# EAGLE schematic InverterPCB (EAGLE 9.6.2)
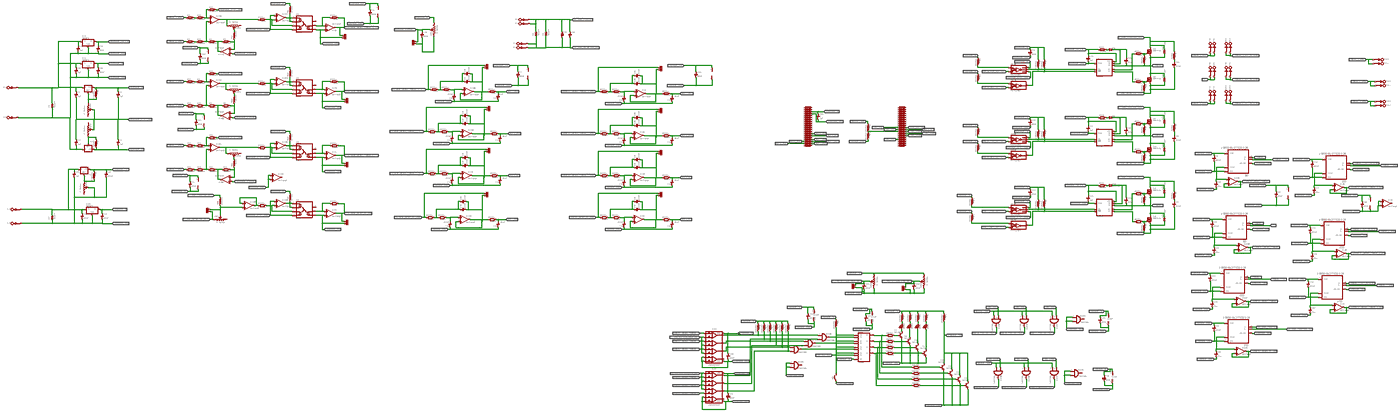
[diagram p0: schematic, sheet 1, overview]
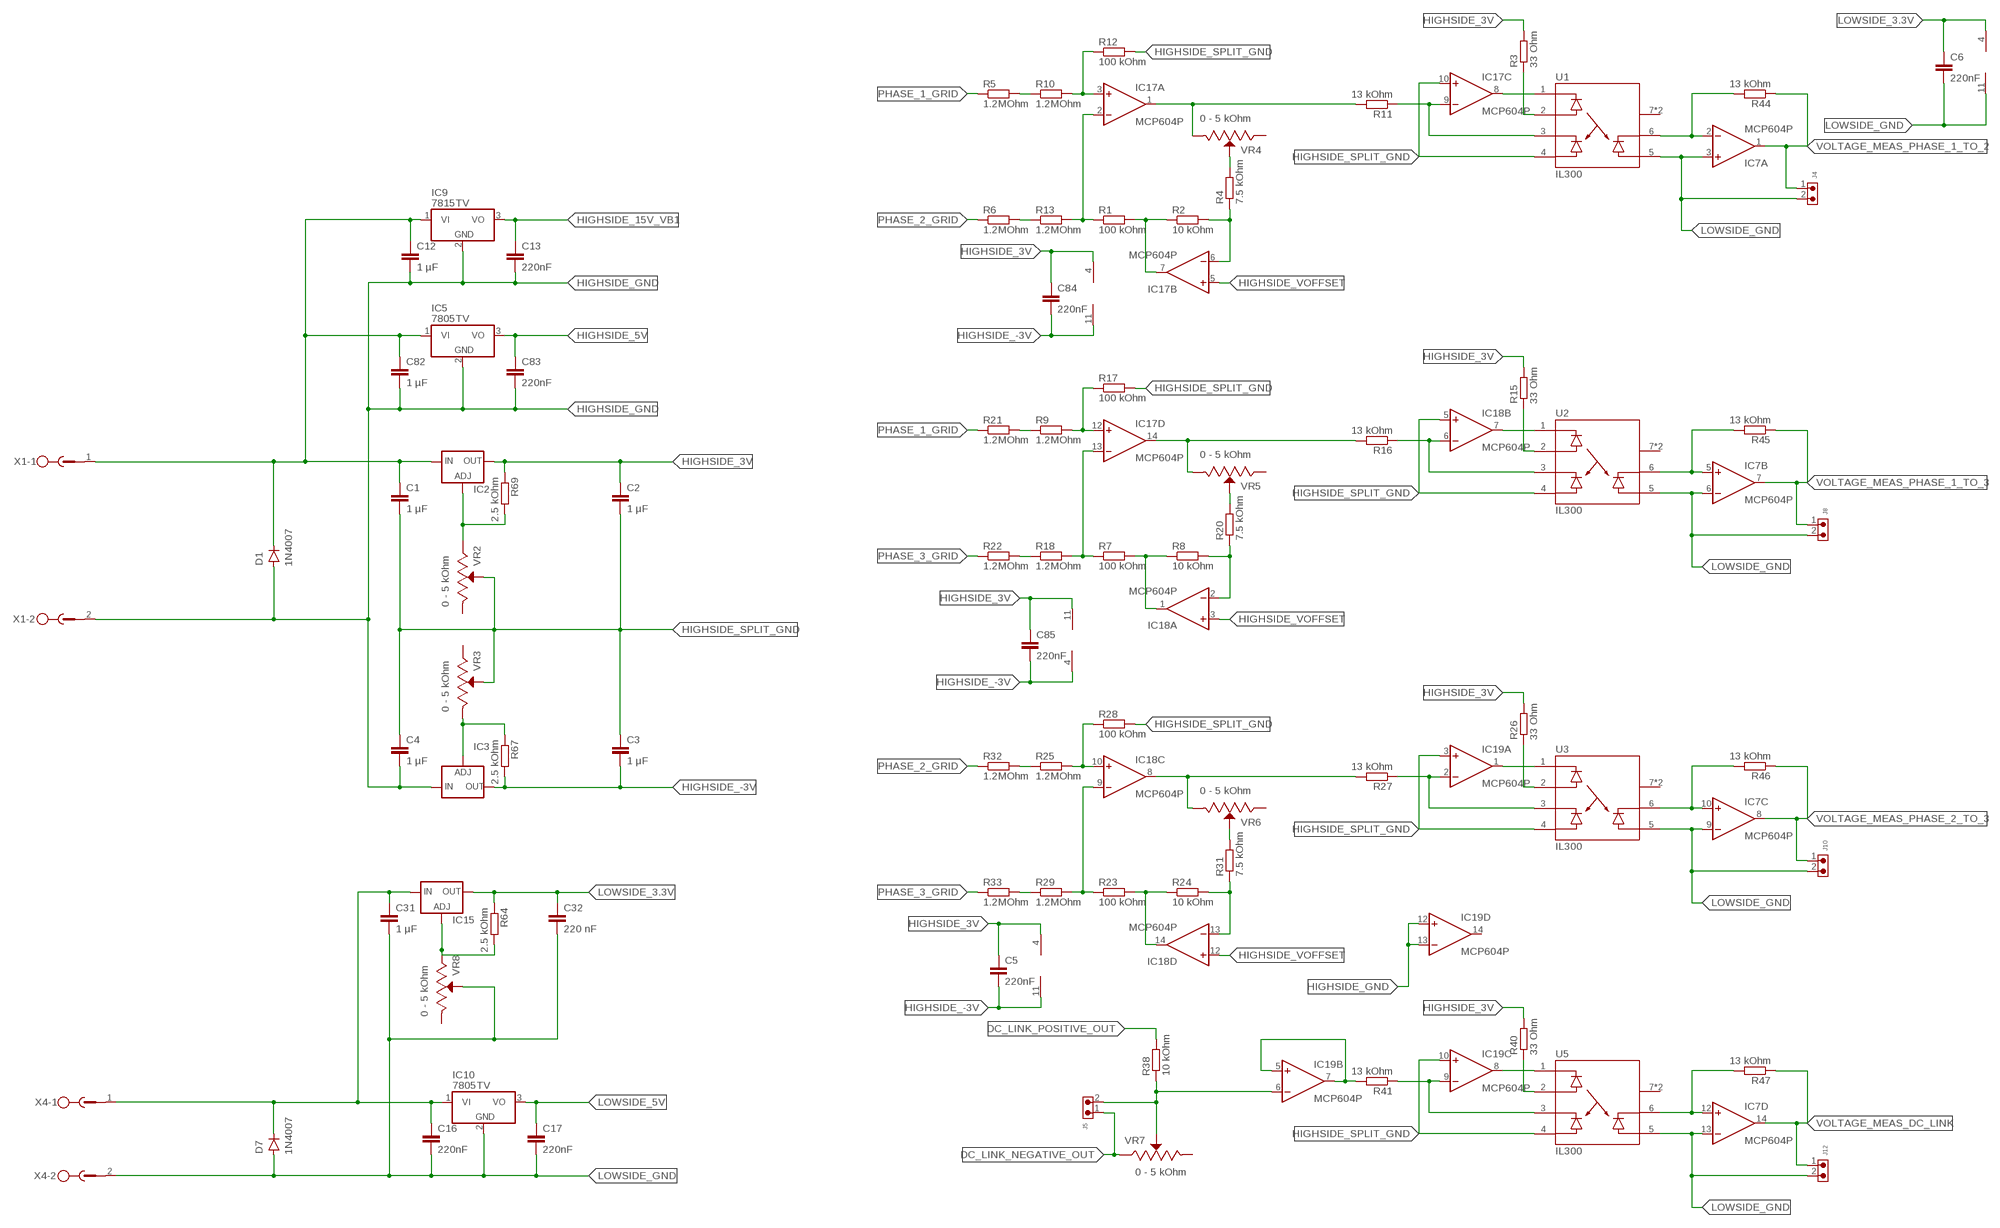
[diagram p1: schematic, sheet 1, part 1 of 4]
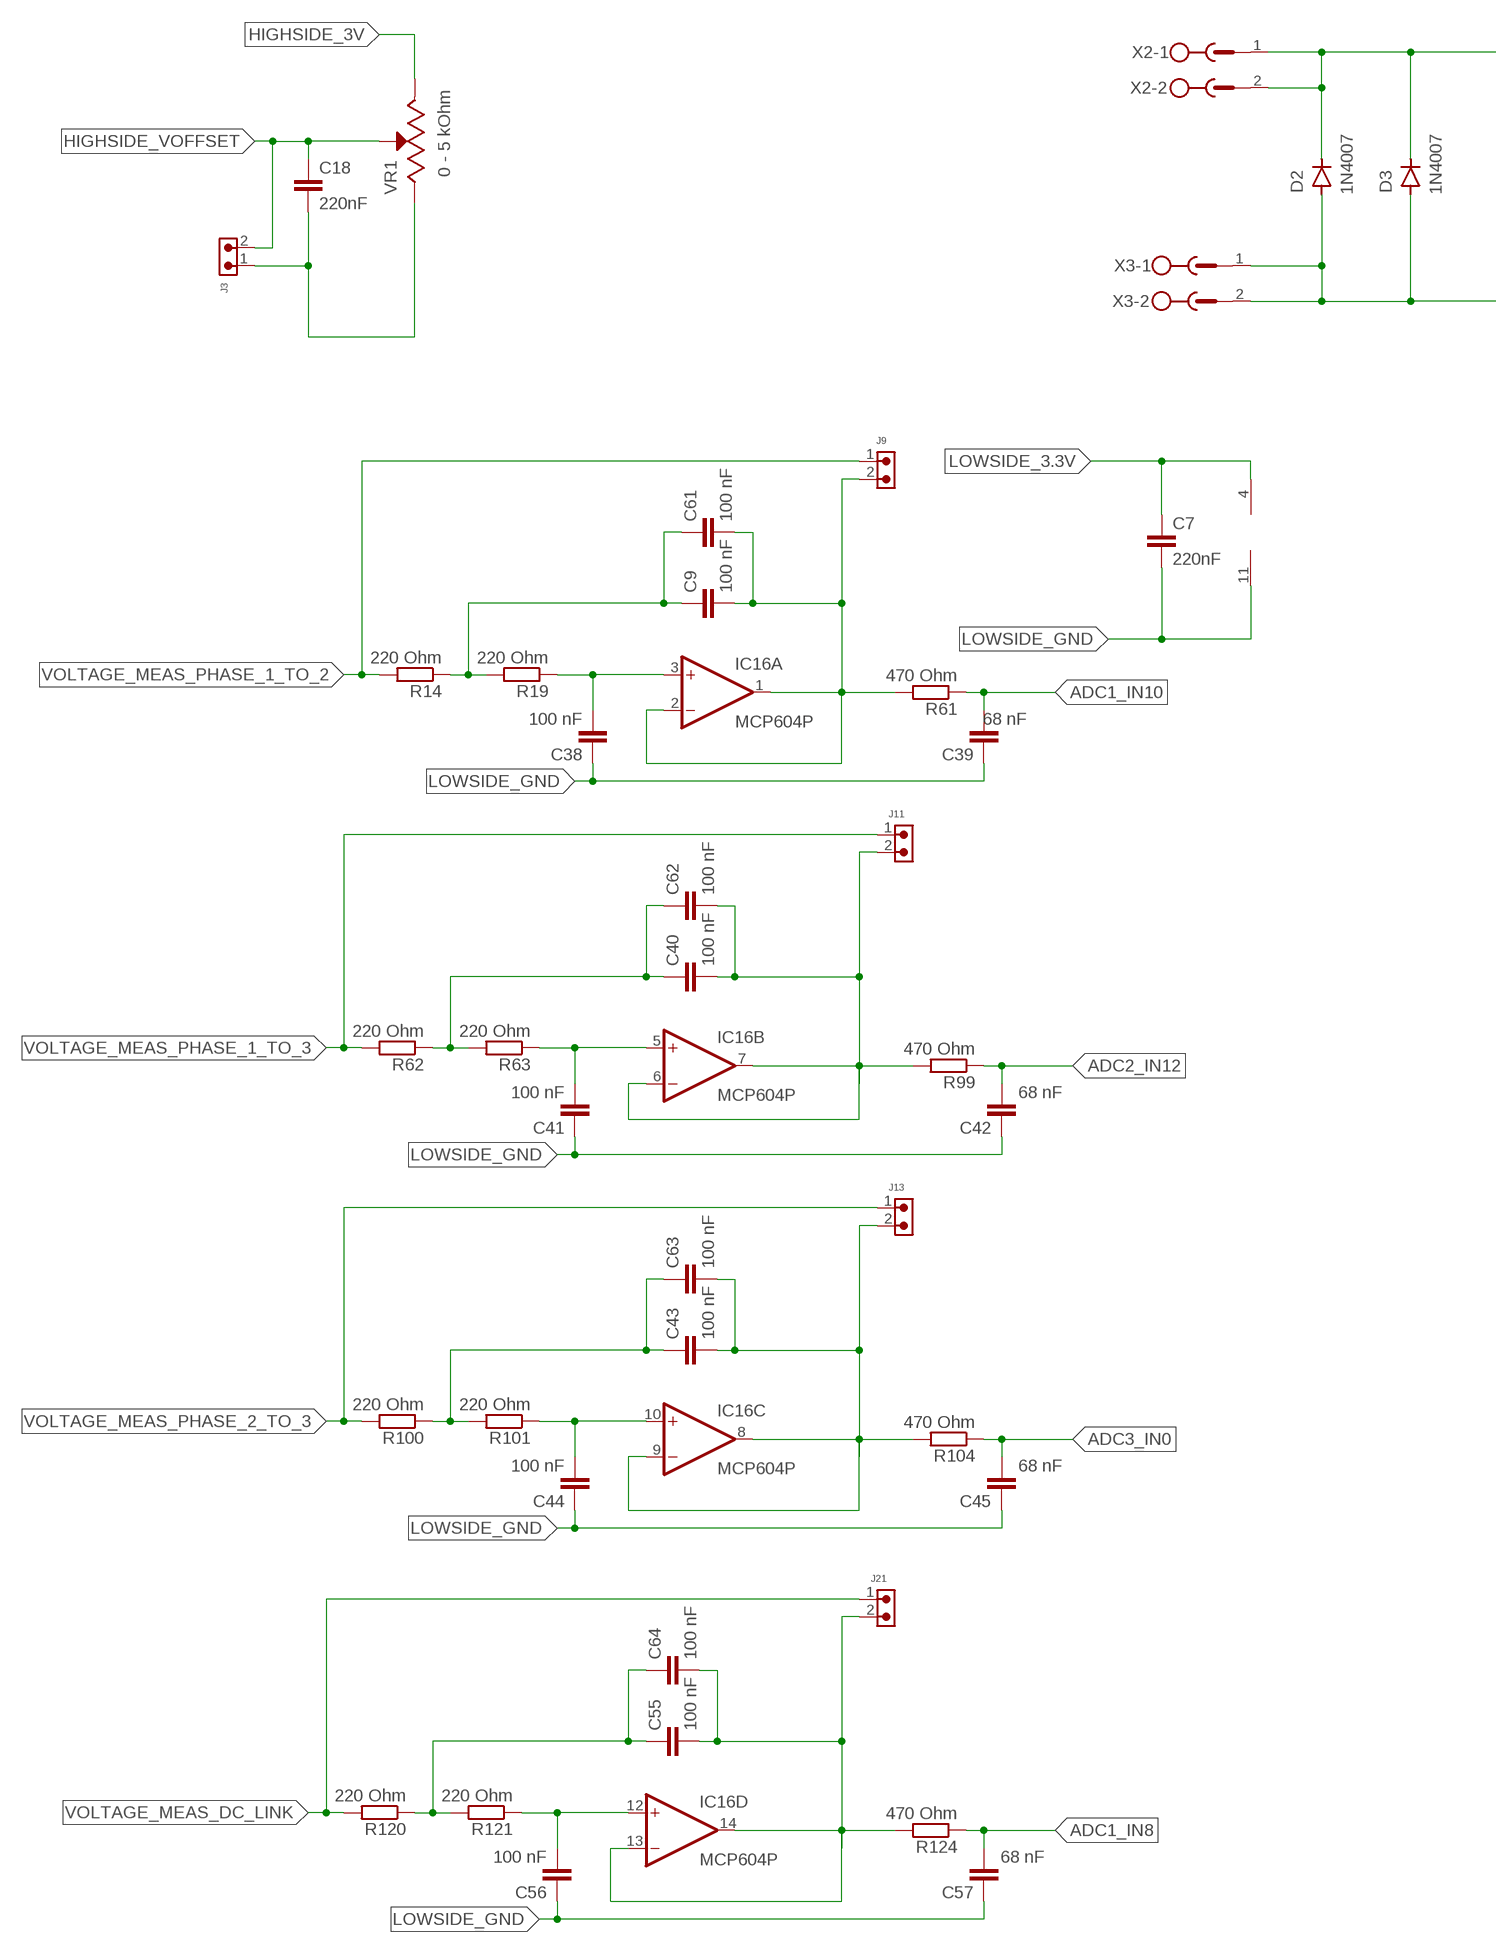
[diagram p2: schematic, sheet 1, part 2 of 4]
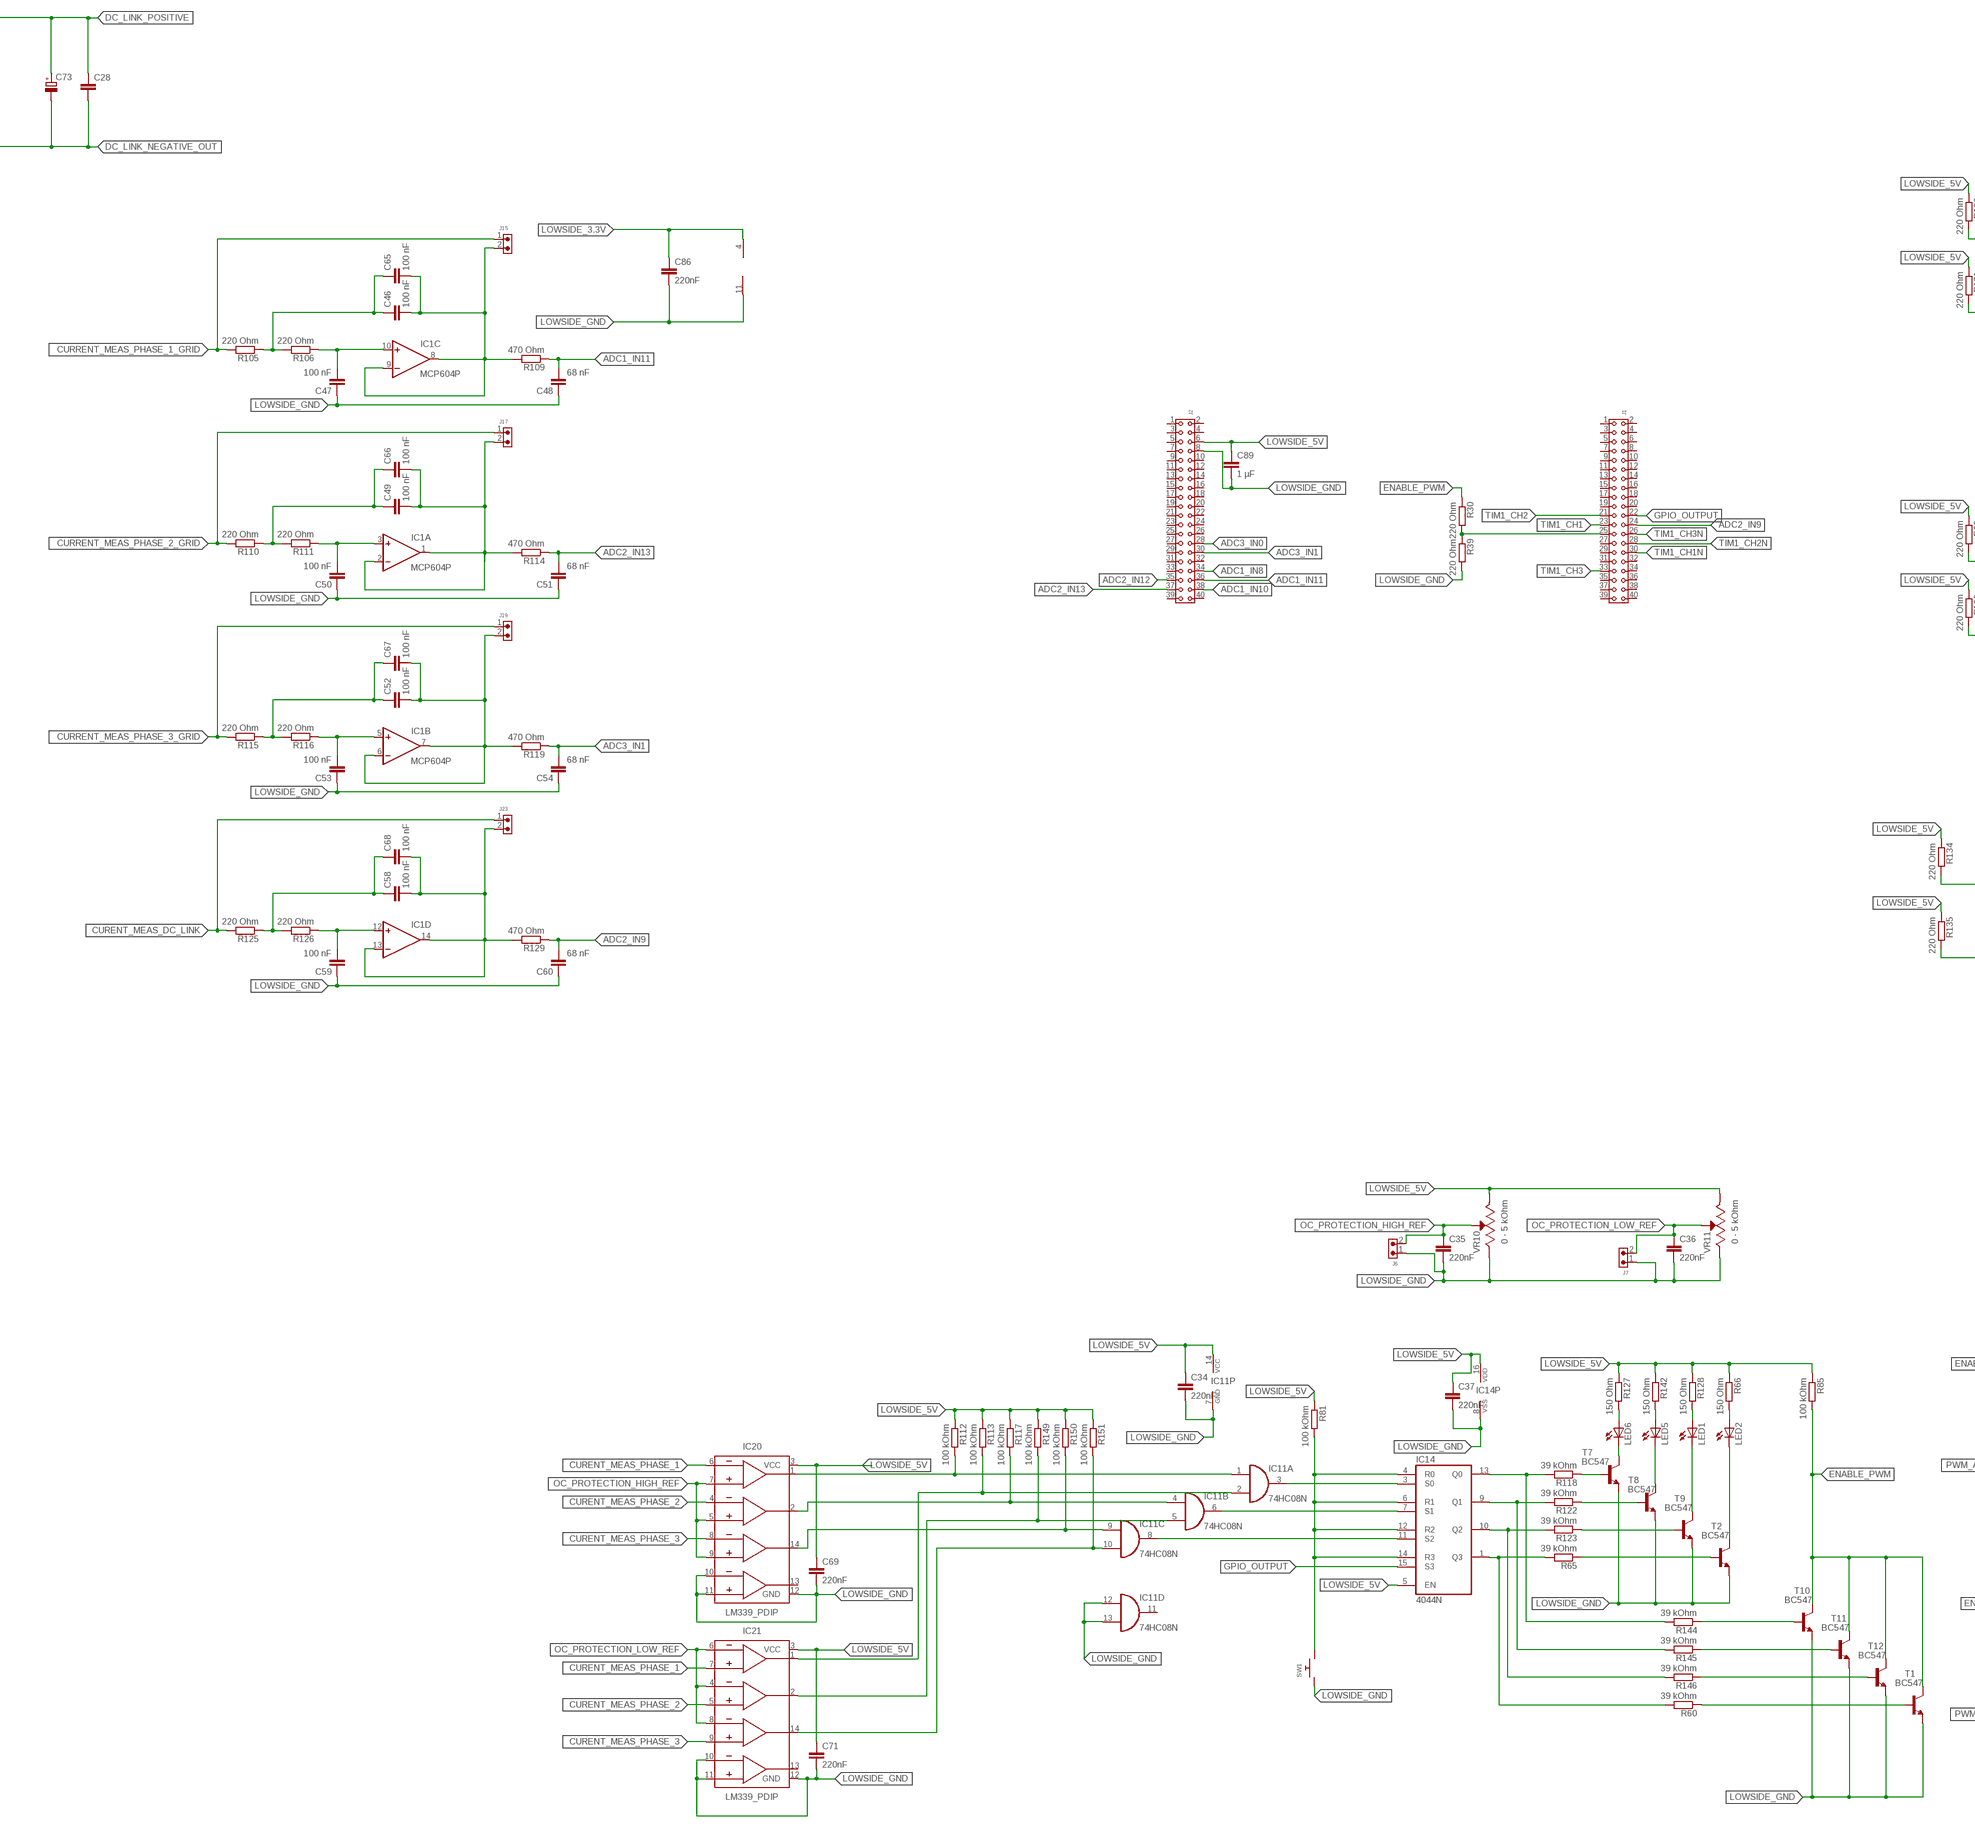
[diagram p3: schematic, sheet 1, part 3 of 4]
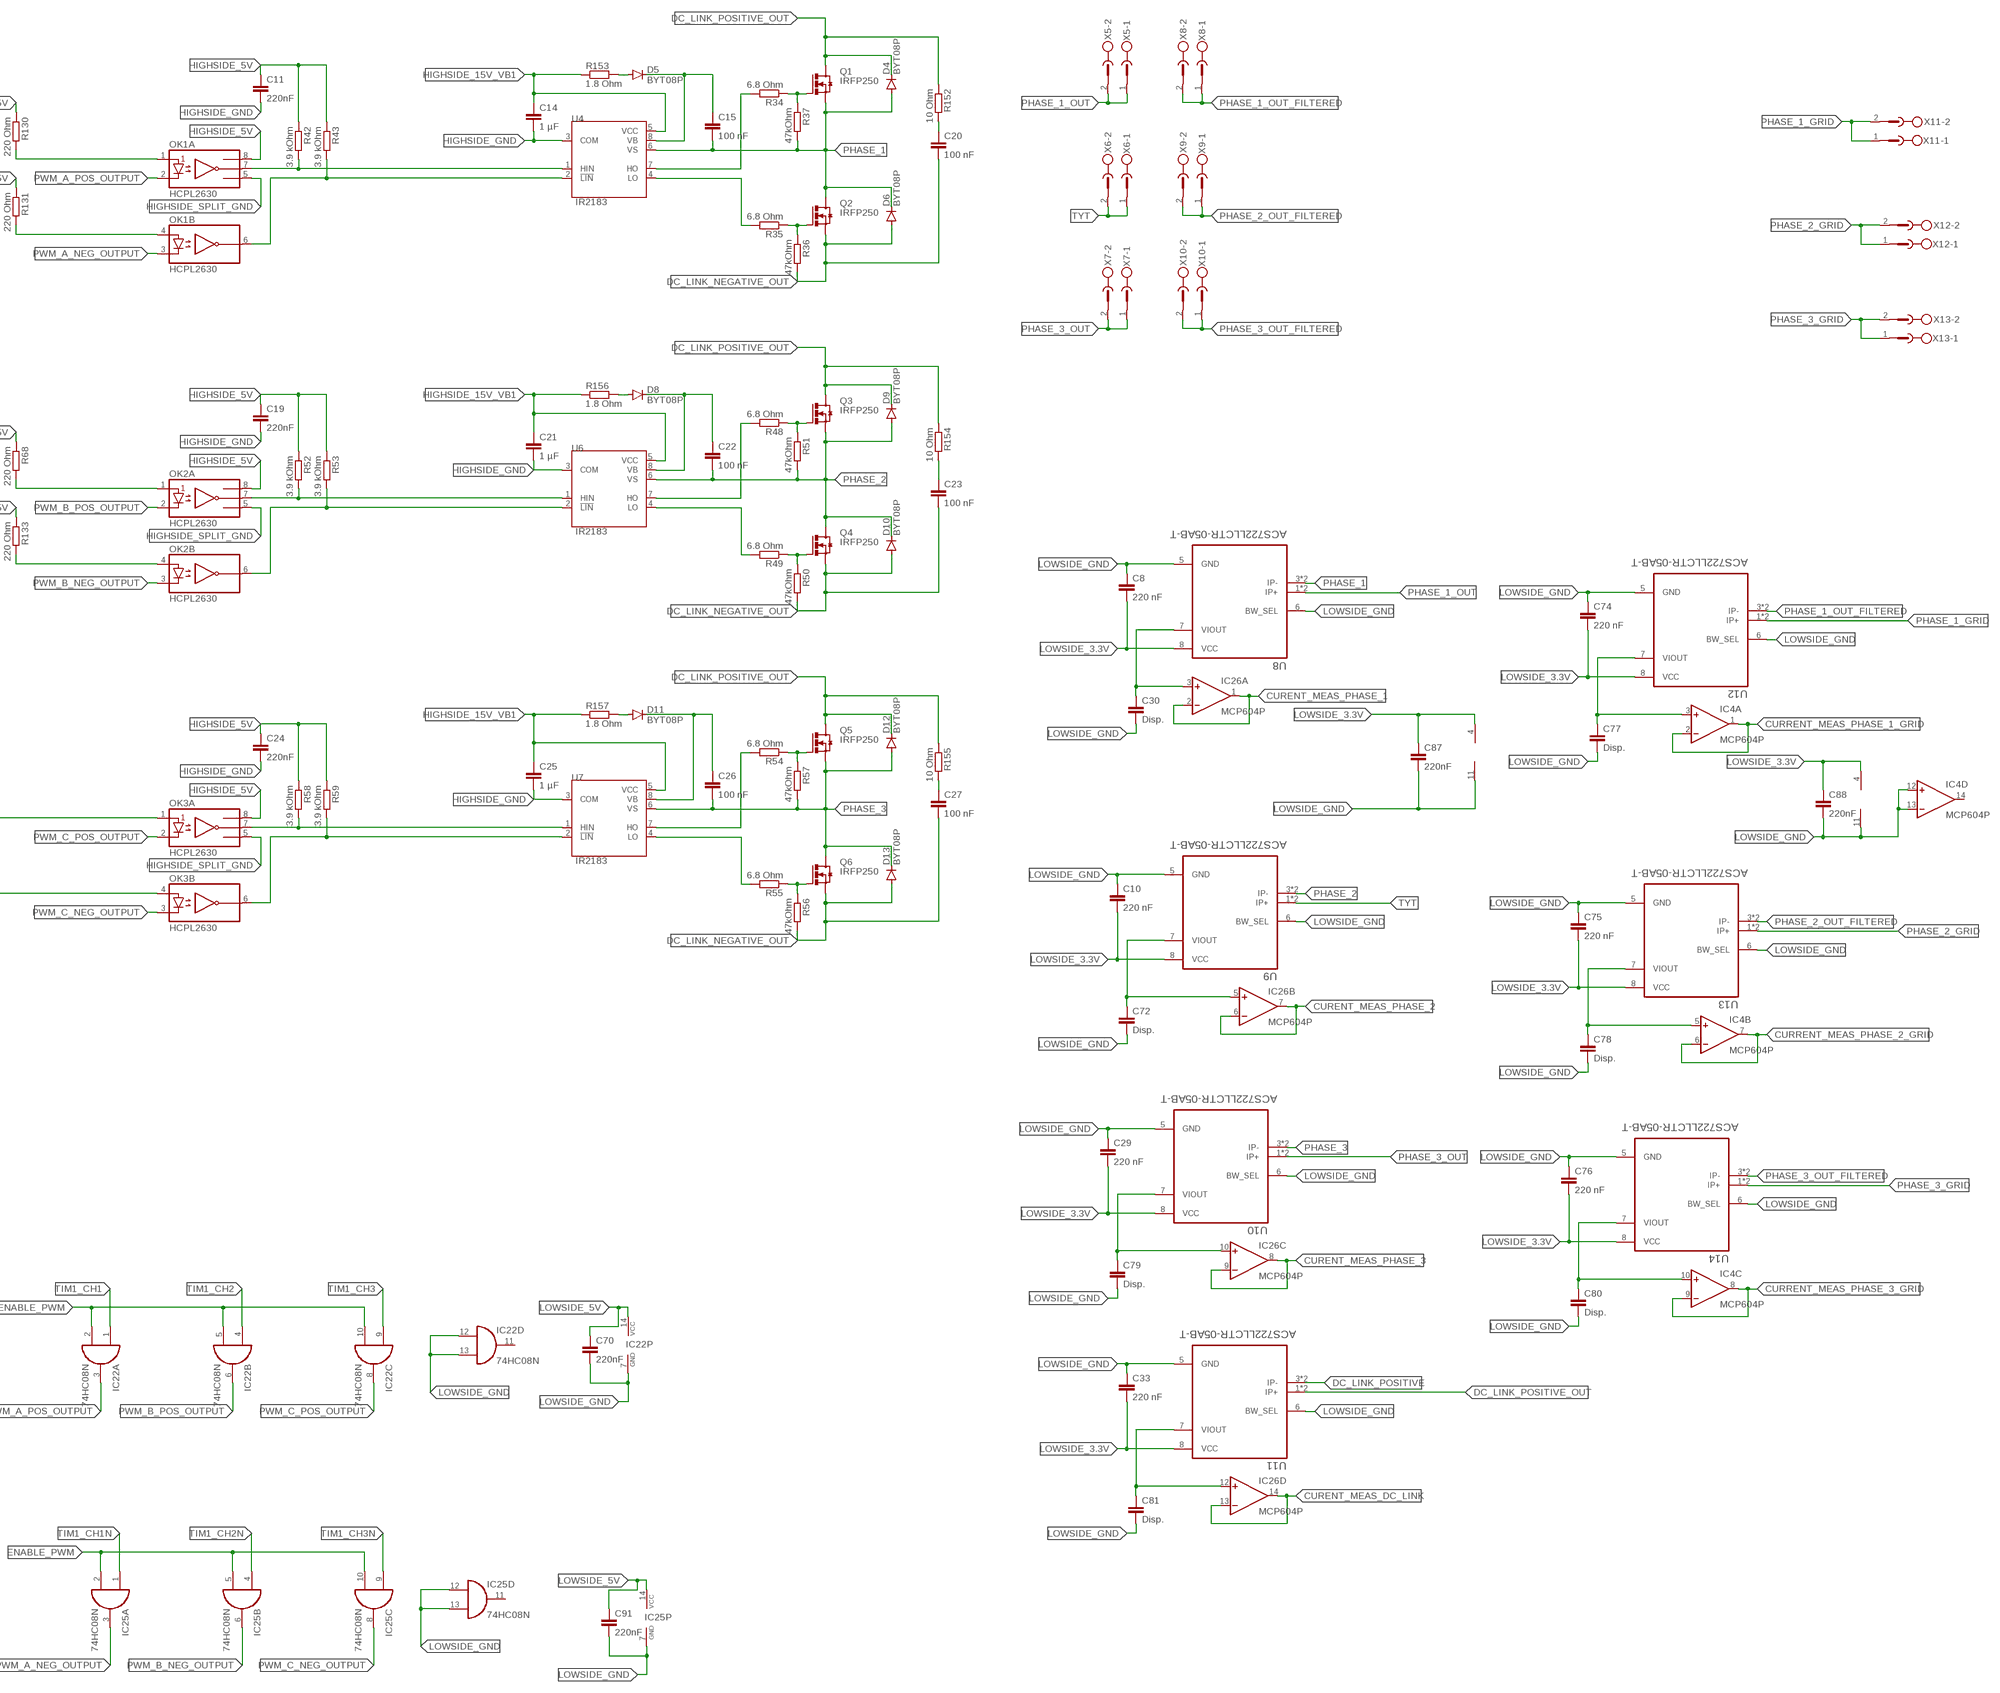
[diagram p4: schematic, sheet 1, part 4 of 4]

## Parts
C1  1 µF  C-EU050-025X075  [C050-025X075]
C2  1 µF  C-EU050-025X075  [C050-025X075]
C3  1 µF  C-EU050-025X075  [C050-025X075]
C4  1 µF  C-EU050-025X075  [C050-025X075]
C5  220nF  C-EU050-025X075  [C050-025X075]
C6  220nF  C-EU050-025X075  [C050-025X075]
C7  220nF  C-EU050-025X075  [C050-025X075]
C8  220 nF  C-EU050-025X075  [C050-025X075]
C9  100 nF  C-EU050-025X075  [C050-025X075]
C10  220 nF  C-EU050-025X075  [C050-025X075]
C11  220nF  C-EU050-025X075  [C050-025X075]
C12  1 µF  C-EU050-025X075  [C050-025X075]
C13  220nF  C-EU050-025X075  [C050-025X075]
C14  1 µF  C-EU050-025X075  [C050-025X075]
C15  100 nF  C-EU050-025X075  [C050-025X075]
C16  220nF  C-EU050-025X075  [C050-025X075]
C17  220nF  C-EU050-025X075  [C050-025X075]
C18  220nF  C-EU050-025X075  [C050-025X075]
C19  220nF  C-EU050-025X075  [C050-025X075]
C20  100 nF  C-EU050-025X075  [C050-025X075]
C21  1 µF  C-EU050-025X075  [C050-025X075]
C22  100 nF  C-EU050-025X075  [C050-025X075]
C23  100 nF  C-EU050-025X075  [C050-025X075]
C24  220nF  C-EU050-025X075  [C050-025X075]
C25  1 µF  C-EU050-025X075  [C050-025X075]
C26  100 nF  C-EU050-025X075  [C050-025X075]
C27  100 nF  C-EU050-025X075  [C050-025X075]
C28  C-EU150-054X183  [C150-054X183]
C29  220 nF  C-EU050-025X075  [C050-025X075]
C30  Disp.  C-EU050-025X075  [C050-025X075]
C31  1 µF  C-EU050-025X075  [C050-025X075]
C32  220 nF  C-EU050-025X075  [C050-025X075]
C33  220 nF  C-EU050-025X075  [C050-025X075]
C34  220nF  C-EU050-025X075  [C050-025X075]
C35  220nF  C-EU050-025X075  [C050-025X075]
C36  220nF  C-EU050-025X075  [C050-025X075]
C37  220nF  C-EU050-025X075  [C050-025X075]
C38  100 nF  C-EU050-025X075  [C050-025X075]
C39  68 nF  C-EU050-025X075  [C050-025X075]
C40  100 nF  C-EU050-025X075  [C050-025X075]
C41  100 nF  C-EU050-025X075  [C050-025X075]
C42  68 nF  C-EU050-025X075  [C050-025X075]
C43  100 nF  C-EU050-025X075  [C050-025X075]
C44  100 nF  C-EU050-025X075  [C050-025X075]
C45  68 nF  C-EU050-025X075  [C050-025X075]
C46  100 nF  C-EU050-025X075  [C050-025X075]
C47  100 nF  C-EU050-025X075  [C050-025X075]
C48  68 nF  C-EU050-025X075  [C050-025X075]
C49  100 nF  C-EU050-025X075  [C050-025X075]
C50  100 nF  C-EU050-025X075  [C050-025X075]
C51  68 nF  C-EU050-025X075  [C050-025X075]
C52  100 nF  C-EU050-025X075  [C050-025X075]
C53  100 nF  C-EU050-025X075  [C050-025X075]
C54  68 nF  C-EU050-025X075  [C050-025X075]
C55  100 nF  C-EU050-025X075  [C050-025X075]
C56  100 nF  C-EU050-025X075  [C050-025X075]
C57  68 nF  C-EU050-025X075  [C050-025X075]
C58  100 nF  C-EU050-025X075  [C050-025X075]
C59  100 nF  C-EU050-025X075  [C050-025X075]
C60  68 nF  C-EU050-025X075  [C050-025X075]
C61  100 nF  C-EU050-025X075  [C050-025X075]
C62  100 nF  C-EU050-025X075  [C050-025X075]
C63  100 nF  C-EU050-025X075  [C050-025X075]
C64  100 nF  C-EU050-025X075  [C050-025X075]
C65  100 nF  C-EU050-025X075  [C050-025X075]
C66  100 nF  C-EU050-025X075  [C050-025X075]
C67  100 nF  C-EU050-025X075  [C050-025X075]
C68  100 nF  C-EU050-025X075  [C050-025X075]
C69  220nF  C-EU050-025X075  [C050-025X075]
C70  220nF  C-EU050-025X075  [C050-025X075]
C71  220nF  C-EU050-025X075  [C050-025X075]
C72  Disp.  C-EU050-025X075  [C050-025X075]
C73  CPOL-EUE7.5-16  [E7,5-16]
C74  220 nF  C-EU050-025X075  [C050-025X075]
C75  220 nF  C-EU050-025X075  [C050-025X075]
C76  220 nF  C-EU050-025X075  [C050-025X075]
C77  Disp.  C-EU050-025X075  [C050-025X075]
C78  Disp.  C-EU050-025X075  [C050-025X075]
C79  Disp.  C-EU050-025X075  [C050-025X075]
C80  Disp.  C-EU050-025X075  [C050-025X075]
C81  Disp.  C-EU050-025X075  [C050-025X075]
C82  1 µF  C-EU050-025X075  [C050-025X075]
C83  220nF  C-EU050-025X075  [C050-025X075]
C84  220nF  C-EU050-025X075  [C050-025X075]
C85  220nF  C-EU050-025X075  [C050-025X075]
C86  220nF  C-EU050-025X075  [C050-025X075]
C87  220nF  C-EU050-025X075  [C050-025X075]
C88  220nF  C-EU050-025X075  [C050-025X075]
C89  1 µF  C-EU050-025X075  [C050-025X075]
C91  220nF  C-EU050-025X075  [C050-025X075]
D1  1N4007  [DO-41]
D2  1N4007  [DO-41]
D3  1N4007  [DO-41]
D4  BYT08P  [TO220ACS]
D5  BYT08P  [TO220ACS]
D6  BYT08P  [TO220ACS]
D7  1N4007  [DO-41]
D8  BYT08P  [TO220ACS]
D9  BYT08P  [TO220ACS]
D10  BYT08P  [TO220ACS]
D11  BYT08P  [TO220ACS]
D12  BYT08P  [TO220ACS]
D13  BYT08P  [TO220ACS]
IC1  MCP604P  [DIL14]
IC2  LM317TS  [317TS]
IC3  LM337TS  [337TS]
IC4  MCP604P  [DIL14]
IC5  7805TV  [TO220V]
IC7  MCP604P  [DIL14]
IC9  7815TV  [TO220V]
IC10  7805TV  [TO220V]
IC11  74HC08N  [DIL14]
IC14  4044N  [DIL16]
IC15  LM317TS  [317TS]
IC16  MCP604P  [DIL14]
IC17  MCP604P  [DIL14]
IC18  MCP604P  [DIL14]
IC19  MCP604P  [DIL14]
IC20  LM339_PDIP  [DIP762W53P254L1969H508Q14B]
IC21  LM339_PDIP  [DIP762W53P254L1969H508Q14B]
IC22  74HC08N  [DIL14]
IC25  74HC08N  [DIL14]
IC26  MCP604P  [DIL14]
J1  6130XX21821_61304021821  [61304021821]
J2  6130XX21821_61304021821  [61304021821]
J3  6130XX11121_61300211121  [61300211121]
J4  6130XX11121_61300211121  [61300211121]
J5  6130XX11121_61300211121  [61300211121]
J6  6130XX11121_61300211121  [61300211121]
J7  6130XX11121_61300211121  [61300211121]
J8  6130XX11121_61300211121  [61300211121]
J9  6130XX11121_61300211121  [61300211121]
J10  6130XX11121_61300211121  [61300211121]
J11  6130XX11121_61300211121  [61300211121]
J12  6130XX11121_61300211121  [61300211121]
J13  6130XX11121_61300211121  [61300211121]
J15  6130XX11121_61300211121  [61300211121]
J17  6130XX11121_61300211121  [61300211121]
J19  6130XX11121_61300211121  [61300211121]
J21  6130XX11121_61300211121  [61300211121]
J23  6130XX11121_61300211121  [61300211121]
LED1  LED3MM  [LED3MM]
LED2  LED3MM  [LED3MM]
LED5  LED3MM  [LED3MM]
LED6  LED3MM  [LED3MM]
OK1  HCPL2630  [DIL08]
OK2  HCPL2630  [DIL08]
OK3  HCPL2630  [DIL08]
Q1  IRFP250  [TO-247AD-V]
Q2  IRFP250  [TO-247AD-V]
Q3  IRFP250  [TO-247AD-V]
Q4  IRFP250  [TO-247AD-V]
Q5  IRFP250  [TO-247AD-V]
Q6  IRFP250  [TO-247AD-V]
R1  100 kOhm  R-EU_0207/10  [0207/10]
R2  10 kOhm  R-EU_0207/10  [0207/10]
R3  33 Ohm  R-EU_0207/10  [0207/10]
R4  7.5 kOhm  R-EU_0207/10  [0207/10]
R5  1.2MOhm  R-EU_0207/10  [0207/10]
R6  1.2MOhm  R-EU_0207/10  [0207/10]
R7  100 kOhm  R-EU_0207/10  [0207/10]
R8  10 kOhm  R-EU_0207/10  [0207/10]
R9  1.2MOhm  R-EU_0207/10  [0207/10]
R10  1.2MOhm  R-EU_0207/10  [0207/10]
R11  13 kOhm  R-EU_0207/10  [0207/10]
R12  100 kOhm  R-EU_0207/10  [0207/10]
R13  1.2MOhm  R-EU_0207/10  [0207/10]
R14  220 Ohm  R-EU_0207/10  [0207/10]
R15  33 Ohm  R-EU_0207/10  [0207/10]
R16  13 kOhm  R-EU_0207/10  [0207/10]
R17  100 kOhm  R-EU_0207/10  [0207/10]
R18  1.2MOhm  R-EU_0207/10  [0207/10]
R19  220 Ohm  R-EU_0207/10  [0207/10]
R20  7.5 kOhm  R-EU_0207/10  [0207/10]
R21  1.2MOhm  R-EU_0207/10  [0207/10]
R22  1.2MOhm  R-EU_0207/10  [0207/10]
R23  100 kOhm  R-EU_0207/10  [0207/10]
R24  10 kOhm  R-EU_0207/10  [0207/10]
R25  1.2MOhm  R-EU_0207/10  [0207/10]
R26  33 Ohm  R-EU_0207/10  [0207/10]
R27  13 kOhm  R-EU_0207/10  [0207/10]
R28  100 kOhm  R-EU_0207/10  [0207/10]
R29  1.2MOhm  R-EU_0207/10  [0207/10]
R30  220 Ohm  R-EU_0207/10  [0207/10]
R31  7.5 kOhm  R-EU_0207/10  [0207/10]
R32  1.2MOhm  R-EU_0207/10  [0207/10]
R33  1.2MOhm  R-EU_0207/10  [0207/10]
R34  6.8 Ohm  R-EU_0207/10  [0207/10]
R35  6.8 Ohm  R-EU_0207/10  [0207/10]
R36  47kOhm  R-EU_0207/10  [0207/10]
R37  47kOhm  R-EU_0207/10  [0207/10]
R38  10 kOhm  R-EU_0207/10  [0207/10]
R39  220 Ohm  R-EU_0207/10  [0207/10]
R40  33 Ohm  R-EU_0207/10  [0207/10]
R41  13 kOhm  R-EU_0207/10  [0207/10]
R42  3.9 kOhm  R-EU_0207/10  [0207/10]
R43  3.9 kOhm  R-EU_0207/10  [0207/10]
R44  13 kOhm  R-EU_0207/10  [0207/10]
R45  13 kOhm  R-EU_0207/10  [0207/10]
R46  13 kOhm  R-EU_0207/10  [0207/10]
R47  13 kOhm  R-EU_0207/10  [0207/10]
R48  6.8 Ohm  R-EU_0207/10  [0207/10]
R49  6.8 Ohm  R-EU_0207/10  [0207/10]
R50  47kOhm  R-EU_0207/10  [0207/10]
R51  47kOhm  R-EU_0207/10  [0207/10]
R52  3.9 kOhm  R-EU_0207/10  [0207/10]
R53  3.9 kOhm  R-EU_0207/10  [0207/10]
R54  6.8 Ohm  R-EU_0207/10  [0207/10]
R55  6.8 Ohm  R-EU_0207/10  [0207/10]
R56  47kOhm  R-EU_0207/10  [0207/10]
R57  47kOhm  R-EU_0207/10  [0207/10]
R58  3.9 kOhm  R-EU_0207/10  [0207/10]
R59  3.9 kOhm  R-EU_0207/10  [0207/10]
R60  39 kOhm  R-EU_0207/10  [0207/10]
R61  470 Ohm  R-EU_0207/10  [0207/10]
R62  220 Ohm  R-EU_0207/10  [0207/10]
R63  220 Ohm  R-EU_0207/10  [0207/10]
R64  2.5 kOhm  R-EU_0207/10  [0207/10]
R65  39 kOhm  R-EU_0207/10  [0207/10]
R66  150 Ohm  R-EU_0207/10  [0207/10]
R67  2.5 kOhm  R-EU_0207/10  [0207/10]
R68  220 Ohm  R-EU_0207/10  [0207/10]
R69  2.5 kOhm  R-EU_0207/10  [0207/10]
R81  100 kOhm  R-EU_0207/10  [0207/10]
R85  100 kOhm  R-EU_0207/10  [0207/10]
R99  470 Ohm  R-EU_0207/10  [0207/10]
R100  220 Ohm  R-EU_0207/10  [0207/10]
R101  220 Ohm  R-EU_0207/10  [0207/10]
R104  470 Ohm  R-EU_0207/10  [0207/10]
R105  220 Ohm  R-EU_0207/10  [0207/10]
R106  220 Ohm  R-EU_0207/10  [0207/10]
R109  470 Ohm  R-EU_0207/10  [0207/10]
R110  220 Ohm  R-EU_0207/10  [0207/10]
R111  220 Ohm  R-EU_0207/10  [0207/10]
R112  100 kOhm  R-EU_0207/10  [0207/10]
R113  100 kOhm  R-EU_0207/10  [0207/10]
R114  470 Ohm  R-EU_0207/10  [0207/10]
R115  220 Ohm  R-EU_0207/10  [0207/10]
R116  220 Ohm  R-EU_0207/10  [0207/10]
R117  100 kOhm  R-EU_0207/10  [0207/10]
R118  39 kOhm  R-EU_0207/10  [0207/10]
R119  470 Ohm  R-EU_0207/10  [0207/10]
R120  220 Ohm  R-EU_0207/10  [0207/10]
R121  220 Ohm  R-EU_0207/10  [0207/10]
R122  39 kOhm  R-EU_0207/10  [0207/10]
R123  39 kOhm  R-EU_0207/10  [0207/10]
R124  470 Ohm  R-EU_0207/10  [0207/10]
R125  220 Ohm  R-EU_0207/10  [0207/10]
R126  220 Ohm  R-EU_0207/10  [0207/10]
R127  150 Ohm  R-EU_0207/10  [0207/10]
R128  150 Ohm  R-EU_0207/10  [0207/10]
R129  470 Ohm  R-EU_0207/10  [0207/10]
R130  220 Ohm  R-EU_0207/10  [0207/10]
R131  220 Ohm  R-EU_0207/10  [0207/10]
R133  220 Ohm  R-EU_0207/10  [0207/10]
R134  220 Ohm  R-EU_0207/10  [0207/10]
R135  220 Ohm  R-EU_0207/10  [0207/10]
R142  150 Ohm  R-EU_0207/10  [0207/10]
R144  39 kOhm  R-EU_0207/10  [0207/10]
R145  39 kOhm  R-EU_0207/10  [0207/10]
R146  39 kOhm  R-EU_0207/10  [0207/10]
R149  100 kOhm  R-EU_0207/10  [0207/10]
R150  100 kOhm  R-EU_0207/10  [0207/10]
R151  100 kOhm  R-EU_0207/10  [0207/10]
R152  10 Ohm  R-EU_0207/10  [0207/10]
R153  1.8 Ohm  R-EU_0207/10  [0207/10]
R154  10 Ohm  R-EU_0207/10  [0207/10]
R155  10 Ohm  R-EU_0207/10  [0207/10]
R156  1.8 Ohm  R-EU_0207/10  [0207/10]
R157  1.8 Ohm  R-EU_0207/10  [0207/10]
SW1  SWITCH_PUSHBUTTONEVQ-PE  [TACT_PANA-EVQ]
T1  BC547  [TO92]
T2  BC547  [TO92]
T7  BC547  [TO92]
T8  BC547  [TO92]
T9  BC547  [TO92]
T10  BC547  [TO92]
T11  BC547  [TO92]
T12  BC547  [TO92]
U1  IL300  [DIP762W52P254L1016H469Q8]
U2  IL300  [DIP762W52P254L1016H469Q8]
U3  IL300  [DIP762W52P254L1016H469Q8]
U4  IR2183  [DIP762W45P254L1092H533Q8]
U5  IL300  [DIP762W52P254L1016H469Q8]
U6  IR2183  [DIP762W45P254L1092H533Q8]
U7  IR2183  [DIP762W45P254L1092H533Q8]
U8  ACS722LLCTR-05AB-T  [SOIC127P600X175-8N]
U9  ACS722LLCTR-05AB-T  [SOIC127P600X175-8N]
U10  ACS722LLCTR-05AB-T  [SOIC127P600X175-8N]
U11  ACS722LLCTR-05AB-T  [SOIC127P600X175-8N]
U12  ACS722LLCTR-05AB-T  [SOIC127P600X175-8N]
U13  ACS722LLCTR-05AB-T  [SOIC127P600X175-8N]
U14  ACS722LLCTR-05AB-T  [SOIC127P600X175-8N]
VR1  0 - 5 kOhm  3296W-1-502LF  [TRIM_3296W-1-502LF]
VR2  0 - 5 kOhm  3296W-1-502LF  [TRIM_3296W-1-502LF]
VR3  0 - 5 kOhm  3296W-1-502LF  [TRIM_3296W-1-502LF]
VR4  0 - 5 kOhm  3296W-1-502LF  [TRIM_3296W-1-502LF]
VR5  0 - 5 kOhm  3296W-1-502LF  [TRIM_3296W-1-502LF]
VR6  0 - 5 kOhm  3296W-1-502LF  [TRIM_3296W-1-502LF]
VR7  0 - 5 kOhm  3296W-1-502LF  [TRIM_3296W-1-502LF]
VR8  0 - 5 kOhm  3296W-1-502LF  [TRIM_3296W-1-502LF]
VR10  0 - 5 kOhm  3296W-1-502LF  [TRIM_3296W-1-502LF]
VR11  0 - 5 kOhm  3296W-1-502LF  [TRIM_3296W-1-502LF]
X1  MSTBV2  [MSTBV2]
X2  MSTBV2  [MSTBV2]
X3  MSTBV2  [MSTBV2]
X4  MSTBV2  [MSTBV2]
X5  MSTBV2  [MSTBV2]
X6  MSTBV2  [MSTBV2]
X7  MSTBV2  [MSTBV2]
X8  MSTBV2  [MSTBV2]
X9  MSTBV2  [MSTBV2]
X10  MSTBV2  [MSTBV2]
X11  MSTBV2  [MSTBV2]
X12  MSTBV2  [MSTBV2]
X13  MSTBV2  [MSTBV2]

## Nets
ADC1_IN8: C57.2 J2.34 R124.1
ADC1_IN10: C39.2 J2.38 R61.1
ADC1_IN11: C48.2 J2.36 R109.1
ADC2_IN9: C60.2 J1.24 R129.1
ADC2_IN12: C42.2 J2.35 R99.1
ADC2_IN13: C51.2 J2.37 R114.1
ADC3_IN0: C45.2 J2.28 R104.1
ADC3_IN1: C54.2 J2.30 R119.1
CURENT_MEAS_DC_LINK: IC26.13(D:-IN) IC26.14(D:OUT) J23.1 R125.2
CURENT_MEAS_PHASE_1: IC20.6(-IN1) IC21.7(+IN1) IC26.1(A:OUT) IC26.2(A:-IN)
CURENT_MEAS_PHASE_2: IC20.4(-IN2) IC21.5(+IN2) IC26.6(B:-IN) IC26.7(B:OUT)
CURENT_MEAS_PHASE_3: IC20.8(-IN3) IC21.9(+IN3) IC26.8(C:OUT) IC26.9(C:-IN)
CURRENT_MEAS_PHASE_1_GRID: IC4.1(A:OUT) IC4.2(A:-IN) J15.1 R105.2
CURRENT_MEAS_PHASE_2_GRID: IC4.6(B:-IN) IC4.7(B:OUT) J17.1 R110.2
CURRENT_MEAS_PHASE_3_GRID: IC4.8(C:OUT) IC4.9(C:-IN) J19.1 R115.2
DC_LINK_NEGATIVE_OUT: C20.2 C23.2 C27.2 C28.2 C73.- D2.A D3.A D6.A D10.A D13.A J5.1 Q2.S Q4.S Q6.S R36.2 R50.2 R56.2 VR7.1(CCW) X3.1 X3.2
DC_LINK_POSITIVE: C28.1 C73.+ D2.C D3.C U11.3(IP-) U11.4(IP-) X2.1 X2.2
DC_LINK_POSITIVE_OUT: D4.C D9.C D12.C Q1.D Q3.D Q5.D R38.2 R152.1 R154.1 R155.1 U11.1(IP+) U11.2(IP+)
DIGITAL_PROTECTION: J1.25 R30.2 R39.1
ENABLE_PWM: IC22.2(A:I1) IC22.5(B:I1) IC22.10(C:I1) IC25.2(A:I1) IC25.5(B:I1) IC25.10(C:I1) R30.1 R85.2 T1.3(C) T10.3(C) T11.3(C) T12.3(C)
GPIO_OUTPUT: IC14.15(S3) J1.22
HIGHSIDE_3V: C2.1 C5.1 C84.1 C85.1 IC2.2(OUT) IC17.4(P:V+) IC18.11(P:V-) IC19.4(P:V+) R3.2 R15.2 R26.2 R40.2 R69.1 VR1.3(CW)
HIGHSIDE_5V: C11.1 C19.1 C24.1 C83.1 IC5.3(VO) OK1.8(A:VCC) OK2.8(A:VCC) OK3.8(A:VCC) R42.1 R43.1 R52.1 R53.1 R58.1 R59.1
HIGHSIDE_15V_VB: C15.1 D5.C U4.8(VB)
HIGHSIDE_15V_VB1: C13.1 C14.1 C21.1 C25.1 IC9.3(VO) R153.1 R156.1 R157.1 U4.5(VCC) U6.5(VCC) U7.5(VCC)
HIGHSIDE_-3V: C3.2 C5.2 C84.2 C85.2 IC3.3(OUT) IC17.11(P:V-) IC18.4(P:V+) IC19.11(P:V-) R67.2
HIGHSIDE_GND [High_gnd]: C4.2 C11.2 C12.2 C13.2 C14.2 C19.2 C21.2 C24.2 C25.2 C82.2 C83.2 D1.A IC3.2(IN) IC5.2(GND) IC9.2(GND) IC19.12(D:+IN) IC19.13(D:-IN) U4.3(COM) U6.3(COM) U7.3(COM) X1.2
HIGHSIDE_LOW_VOLTAGE_INPUT: C1.1 C12.1 C82.1 D1.C IC2.3(IN) IC5.1(VI) IC9.1(VI) X1.1
HIGHSIDE_SPLIT_GND: C1.2 C2.2 C3.1 C4.1 IC17.10(C:+IN) IC18.5(B:+IN) IC19.3(A:+IN) IC19.10(C:+IN) OK1.5(A:GND) OK2.5(A:GND) OK3.5(A:GND) R12.2 R17.2 R28.2 U1.4(A1) U2.4(A1) U3.4(A1) U5.4(A1) VR2.2(WIPER) VR3.2(WIPER)
HIGHSIDE_VOFFSET: C18.1 IC17.5(B:+IN) IC18.3(A:+IN) IC18.12(D:+IN) J3.2 VR1.2(WIPER)
LACH_RESET: IC14.4(R0) IC14.6(R1) IC14.12(R2) IC14.14(R3) R81.2 SW1.P$2
LOWSIDE_3.3V: C6.1 C7.1 C8.2 C10.2 C29.2 C32.1 C33.2 C74.2 C75.2 C76.2 C86.1 C87.1 C88.1 IC1.4(P:V+) IC4.4(P:V+) IC7.4(P:V+) IC15.2(OUT) IC16.4(P:V+) IC26.4(P:V+) R64.1 U8.8(VCC) U9.8(VCC) U10.8(VCC) U11.8(VCC) U12.8(VCC) U13.8(VCC) U14.8(VCC)
LOWSIDE_5V: C17.1 C34.1 C37.1 C69.1 C70.1 C71.1 C89.1 C91.1 IC10.3(VO) IC11.14(P:VCC) IC14.5(EN) IC14.16(VDD) IC20.3(VCC) IC21.3(VCC) IC22.14(P:VCC) IC25.14(P:VCC) J2.6 R66.1 R68.1 R81.1 R85.1 R112.1 R113.1 R117.1 R127.1 R128.1 R130.1 R131.1 R133.1 R134.1 R135.1 R142.1 R149.1 R150.1 R151.1 VR10.3(CW) VR11.3(CW)
LOWSIDE_GND [low_gnd]: C6.2 C7.2 C8.1 C10.1 C16.2 C17.2 C29.1 C30.2 C31.2 C32.2 C33.1 C34.2 C35.2 C36.2 C37.2 C38.1 C39.1 C41.1 C42.1 C44.1 C45.1 C47.1 C48.1 C50.1 C51.1 C53.1 C54.1 C56.1 C57.1 C59.1 C60.1 C69.2 C70.2 C71.2 C72.2 C74.1 C75.1 C76.1 C77.2 C78.2 C79.2 C80.2 C81.2 C86.2 C87.2 C88.2 C89.2 C91.2 D7.A IC1.11(P:V-) IC4.11(P:V-) IC4.12(D:+IN) IC4.13(D:-IN) IC7.3(A:+IN) IC7.6(B:-IN) IC7.9(C:-IN) IC7.11(P:V-) IC7.13(D:-IN) IC10.2(GND) IC11.7(P:GND) IC11.12(D:I0) IC11.13(D:I1) IC14.8(VSS) IC16.11(P:V-) IC20.10(-IN4) IC20.11(+IN4) IC20.12(GND) IC21.10(-IN4) IC21.11(+IN4) IC21.12(GND) IC22.7(P:GND) IC22.12(D:I0) IC22.13(D:I1) IC25.7(P:GND) IC25.12(D:I0) IC25.13(D:I1) IC26.11(P:V-) J2.8 J4.2 J6.1 J7.1 J8.2 J10.2 J12.2 R39.2 SW1.P$1 T1.1(E) T2.1(E) T7.1(E) T8.1(E) T9.1(E) T10.1(E) T11.1(E) T12.1(E) U1.5(A2) U2.5(A2) U3.5(A2) U5.5(A2) U8.5(GND) U8.6(BW_SEL) U9.5(GND) U9.6(BW_SEL) U10.5(GND) U10.6(BW_SEL) U11.5(GND) U11.6(BW_SEL) U12.5(GND) U12.6(BW_SEL) U13.5(GND) U13.6(BW_SEL) U14.5(GND) U14.6(BW_SEL) VR8.2(WIPER) VR10.1(CCW) VR11.1(CCW) X4.2
N$1: IC17.8(C:OUT) U1.1(C3)
N$2: R3.1 U1.2(A3)
N$3: IC17.2(A:-IN) R1.1 R13.2
N$4: IC17.9(C:-IN) R11.1 U1.3(C1)
N$5: R4.2 VR4.2(WIPER)
N$6: IC17.1(A:OUT) R11.2 VR4.3(CW)
N$7: IC17.7(B:OUT) R1.2 R2.1
N$8: IC17.3(A:+IN) R10.2 R12.1
N$9: IC17.6(B:-IN) R2.2 R4.1
N$10: R5.2 R10.1
N$11: R6.2 R13.1
N$12: IC18.7(B:OUT) U2.1(C3)
N$13: R15.1 U2.2(A3)
N$14: IC18.6(B:-IN) R16.1 U2.3(C1)
N$15: IC17.14(D:OUT) R16.2 VR5.3(CW)
N$16: IC17.12(D:+IN) R9.2 R17.1
N$17: IC17.13(D:-IN) R7.1 R18.2
N$18: IC18.1(A:OUT) R7.2 R8.1
N$19: IC18.2(A:-IN) R8.2 R20.1
N$20: R20.2 VR5.2(WIPER)
N$21: R9.1 R21.2
N$22: R18.1 R22.2
N$23: IC19.1(A:OUT) U3.1(C3)
N$24: R26.1 U3.2(A3)
N$25: IC19.2(A:-IN) R27.1 U3.3(C1)
N$26: IC18.8(C:OUT) R27.2 VR6.3(CW)
N$27: IC18.10(C:+IN) R25.2 R28.1
N$28: IC18.9(C:-IN) R23.1 R29.2
N$29: IC18.14(D:OUT) R23.2 R24.1
N$30: IC18.13(D:-IN) R24.2 R31.1
N$31: R31.2 VR6.2(WIPER)
N$32: R25.1 R32.2
N$33: R29.1 R33.2
N$34: R60.1 T1.2(B)
N$35: IC15.1(ADJ) R64.2 VR8.1(CCW)
N$36: D5.A R153.2
N$37: C16.1 C31.1 D7.C IC10.1(VI) IC15.3(IN) X4.1
N$38: IC19.6(B:-IN) J5.2 R38.1 VR7.2(WIPER)
N$39: R40.1 U5.2(A3)
N$40: Q1.G R34.1 R37.1
N$41: OK1.7(A:VO1) R42.2 U4.1(HIN)
N$42: Q2.G R35.1 R36.1
N$43: IC7.2(A:-IN) R44.2 U1.6(C2)
N$44: OK1.6(B:VO2) R43.2 U4.2(!LIN)
N$45: R35.2 U4.4(LO)
N$46: R34.2 U4.7(HO)
N$47: IC19.8(C:OUT) U5.1(C3)
N$48: IC19.9(C:-IN) R41.1 U5.3(C1)
N$49: C22.1 D8.C U6.8(VB)
N$50: IC7.5(B:+IN) R45.2 U2.6(C2)
N$51: IC14.1(Q3) R60.2 R65.2
N$52: C30.1 IC26.3(A:+IN) U8.7(VIOUT)
N$53: C26.1 D11.C U7.8(VB)
N$54: IC19.5(B:+IN) IC19.7(B:OUT) R41.2
N$55: C72.1 IC26.5(B:+IN) U9.7(VIOUT)
N$56: IC7.10(C:+IN) R46.2 U3.6(C2)
N$57: IC3.1(ADJ) R67.1 VR3.3(CW)
N$58: IC2.1(ADJ) R69.2 VR2.1(CCW)
N$59: C77.1 IC4.3(A:+IN) U12.7(VIOUT)
N$60: IC7.12(D:+IN) R47.2 U5.6(C2)
N$61: R65.1 T2.2(B)
N$63: C81.1 IC26.12(D:+IN) U11.7(VIOUT)
N$64: LED2.A R66.2
N$65: Q3.G R48.1 R51.1
N$66: Q4.G R49.1 R50.1
N$67: OK2.7(A:VO1) R52.2 U6.1(HIN)
N$68: OK2.6(B:VO2) R53.2 U6.2(!LIN)
N$69: R48.2 U6.7(HO)
N$70: R49.2 U6.4(LO)
N$71: D8.A R156.2
N$74: Q5.G R54.1 R57.1
N$75: Q6.G R55.1 R56.1
N$76: OK3.7(A:VO1) R58.2 U7.1(HIN)
N$77: OK3.6(B:VO2) R59.2 U7.2(!LIN)
N$78: R54.2 U7.7(HO)
N$79: R55.2 U7.4(LO)
N$80: D11.A R157.2
N$84: C38.2 IC16.3(A:+IN) R19.1
N$86: C9.1 C61.1 R14.1 R19.2
N$87: C78.1 IC4.5(B:+IN) U13.7(VIOUT)
N$88: C41.2 IC16.5(B:+IN) R63.1
N$89: LED2.K(C) T2.3(C)
N$90: C40.1 C62.1 R62.1 R63.2
N$91: IC11.3(A:O) IC14.3(S0)
N$93: C79.1 IC26.10(C:+IN) U10.7(VIOUT)
N$94: C44.2 IC16.10(C:+IN) R101.1
N$95: C43.1 C63.1 R100.1 R101.2
N$96: C80.1 IC4.10(C:+IN) U14.7(VIOUT)
N$99: C47.2 IC1.10(C:+IN) R106.1
N$100: C46.1 C65.1 R105.1 R106.2
N$104: C50.2 IC1.3(A:+IN) R111.1
N$105: C49.1 C66.1 R110.1 R111.2
N$106: IC11.6(B:O) IC14.7(S1)
N$107: IC11.8(C:O) IC14.11(S2)
N$108: LED6.A R127.2
N$109: C53.2 IC1.5(B:+IN) R116.1
N$110: C52.1 C67.1 R115.1 R116.2
N$111: LED5.A R142.2
N$112: LED1.A R128.2
N$113: LED1.K(C) T9.3(C)
N$114: C56.2 IC16.12(D:+IN) R121.1
N$115: C55.1 C64.1 R120.1 R121.2
N$116: LED5.K(C) T8.3(C)
N$117: LED6.K(C) T7.3(C)
N$119: C59.2 IC1.12(D:+IN) R126.1
N$120: C58.1 C68.1 R125.1 R126.2
N$121: OK1.1(A:A1) R130.2
N$122: OK1.4(B:A2) R131.2
N$123: OK2.1(A:A1) R68.2
N$124: OK2.4(B:A2) R133.2
N$125: OK3.1(A:A1) R134.2
N$126: OK3.4(B:A2) R135.2
N$127: R118.1 T7.2(B)
N$128: R122.1 T8.2(B)
N$129: R123.1 T9.2(B)
N$130: IC14.13(Q0) R118.2 R144.2
N$131: IC14.9(Q1) R122.2 R145.2
N$132: IC14.10(Q2) R123.2 R146.2
N$142: R144.1 T10.2(B)
N$143: R145.1 T11.2(B)
N$144: R146.1 T12.2(B)
N$151: IC11.2(A:I1) IC21.1(OUT1) R113.2
N$152: IC11.5(B:I1) IC21.2(OUT2) R149.2
N$153: IC11.10(C:I1) IC21.14(OUT3) R151.2
N$154: IC11.1(A:I0) IC20.1(OUT1) R112.2
N$155: IC11.4(B:I0) IC20.2(OUT2) R117.2
N$156: IC11.9(C:I0) IC20.14(OUT3) R150.2
N$157: C18.2 J3.1 VR1.1(CCW)
N$158: C20.1 R152.2
N$163: C23.1 R154.2
N$164: C27.1 R155.2
NO: C9.2 C61.2 IC16.1(A:OUT) IC16.2(A:-IN) J9.2 R61.2
NO1: C40.2 C62.2 IC16.6(B:-IN) IC16.7(B:OUT) J11.2 R99.2
NO2: C43.2 C63.2 IC16.8(C:OUT) IC16.9(C:-IN) J13.2 R104.2
NO3: C46.2 C65.2 IC1.8(C:OUT) IC1.9(C:-IN) J15.2 R109.2
NO4: C49.2 C66.2 IC1.1(A:OUT) IC1.2(A:-IN) J17.2 R114.2
NO5: C52.2 C67.2 IC1.6(B:-IN) IC1.7(B:OUT) J19.2 R119.2
NO6: C55.2 C64.2 IC16.13(D:-IN) IC16.14(D:OUT) J21.2 R124.2
NO7: C58.2 C68.2 IC1.13(D:-IN) IC1.14(D:OUT) J23.2 R129.2
OC_PROTECTION_HIGH_REF: C35.1 IC20.5(+IN2) IC20.7(+IN1) IC20.9(+IN3) J6.2 VR10.2(WIPER)
OC_PROTECTION_LOW_REF: C36.1 IC21.4(-IN2) IC21.6(-IN1) IC21.8(-IN3) J7.2 VR11.2(WIPER)
PHASE_1: C15.2 D4.A D6.C Q1.S Q2.D R37.2 U4.6(VS) U8.3(IP-) U8.4(IP-)
PHASE_1_GRID: R5.1 R21.1 U12.1(IP+) U12.2(IP+) X11.1 X11.2
PHASE_1_OUT: U8.1(IP+) U8.2(IP+) X5.1 X5.2
PHASE_1_OUT_FILTERED: U12.3(IP-) U12.4(IP-) X8.1 X8.2
PHASE_2: C22.2 D9.A D10.C Q3.S Q4.D R51.2 U6.6(VS) U9.3(IP-) U9.4(IP-)
PHASE_2_GRID: R6.1 R32.1 U13.1(IP+) U13.2(IP+) X12.1 X12.2
PHASE_2_OUT_FILTERED: U13.3(IP-) U13.4(IP-) X9.1 X9.2
PHASE_3: C26.2 D12.A D13.C Q5.S Q6.D R57.2 U7.6(VS) U10.3(IP-) U10.4(IP-)
PHASE_3_GRID: R22.1 R33.1 U14.1(IP+) U14.2(IP+) X13.1 X13.2
PHASE_3_OUT: U10.1(IP+) U10.2(IP+) X7.1 X7.2
PHASE_3_OUT_FILTERED: U14.3(IP-) U14.4(IP-) X10.1 X10.2
PWM_A_NEG_OUTPUT: IC25.3(A:O) OK1.3(B:C2)
PWM_A_POS_OUTPUT: IC22.3(A:O) OK1.2(A:C1)
PWM_B_NEG_OUTPUT: IC25.6(B:O) OK2.3(B:C2)
PWM_B_POS_OUTPUT: IC22.6(B:O) OK2.2(A:C1)
PWM_C_NEG_OUTPUT: IC25.8(C:O) OK3.3(B:C2)
PWM_C_POS_OUTPUT: IC22.8(C:O) OK3.2(A:C1)
TIM1_CH1: IC22.1(A:I0) J1.23
TIM1_CH1N: IC25.1(A:I0) J1.30
TIM1_CH2: IC22.4(B:I0) J1.21
TIM1_CH2N: IC25.4(B:I0) J1.28
TIM1_CH3: IC22.9(C:I0) J1.33
TIM1_CH3N: IC25.9(C:I0) J1.26
TYT: U9.1(IP+) U9.2(IP+) X6.1 X6.2
VOLTAGE_MEAS_DC_LINK: IC7.14(D:OUT) J12.1 J21.1 R47.1 R120.2
VOLTAGE_MEAS_PHASE_1_TO_2: IC7.1(A:OUT) J4.1 J9.1 R14.2 R44.1
VOLTAGE_MEAS_PHASE_1_TO_3: IC7.7(B:OUT) J8.1 J11.1 R45.1 R62.2
VOLTAGE_MEAS_PHASE_2_TO_3: IC7.8(C:OUT) J10.1 J13.1 R46.1 R100.2
Unconnected: IC4.14(D:OUT) IC11.11(D:O) IC19.14(D:OUT) IC20.13(OUT4) IC21.13(OUT4) IC22.11(D:O) IC25.11(D:O) J1.1 J1.2 J1.3 J1.4 J1.5 J1.6 J1.7 J1.8 J1.9 J1.10 J1.11 J1.12 J1.13 J1.14 J1.15 J1.16 J1.17 J1.18 J1.19 J1.20 J1.27 J1.29 J1.31 J1.32 J1.34 J1.35 J1.36 J1.37 J1.38 J1.39 J1.40 J2.1 J2.2 J2.3 J2.4 J2.5 J2.7 J2.9 J2.10 J2.11 J2.12 J2.13 J2.14 J2.15 J2.16 J2.17 J2.18 J2.19 J2.20 J2.21 J2.22 J2.23 J2.24 J2.25 J2.26 J2.27 J2.29 J2.31 J2.32 J2.33 J2.39 J2.40 U1.7(NC) U1.8(NC) U2.7(NC) U2.8(NC) U3.7(NC) U3.8(NC) U5.7(NC) U5.8(NC) VR2.3(CW) VR3.1(CCW) VR4.1(CCW) VR5.1(CCW) VR6.1(CCW) VR7.3(CW) VR8.3(CW)

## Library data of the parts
C1-C72 C74-C89 C91 = rcl:C-EU: CAPACITOR, European symbol; SPICEPREFIX: C
C73 = rcl:CPOL-EU: POLARIZED CAPACITOR, European symbol; SPICEPREFIX: C
D1-D3 D7 = Diodes:1N4007: DIODE GEN PURP 1KV 1A DO41; CREATED_BY: PCBLayout.com; DIGIKEY_PART_NUMBER: 1N4007MSCT-ND; MANUFACTURER: Micro Commercial Co; MPN: 1N4007; PACKAGE: DO-41
D4-D6 D8-D13 = diode:BYT08P: DIODE
IC1 IC4 IC7 IC16-IC19 IC26 = linear:MCP604: Quad Op Amp 2.7V to 6.0V Single Supply CMOS Source: http://ww1.microchip.com/downloads/en/DeviceDoc/21314g.pdf
IC2 IC15 = v-reg:LM317TS: VOLTAGE REGULATOR
IC3 = v-reg:LM337TS: VOLTAGE REGULATOR
IC5 IC9 IC10 = linear:78*: Positive VOLTAGE REGULATOR Source: http://cache.national.com/ds/LM/LM78L05.pdf http://www.fairchildsemi.com/ds/LM/LM7805.pdf
IC11 IC22 IC25 = 74xx-eu:74*08: Quad 2-input AND gate
IC14 = 40xx:4044: Quad 3-state NAND R/S LATCH
IC20 IC21 = Tinkercad:LM339: Quad Comparators Reference Datasheet
J1 J2 = Wurth_Connectors_WR-PHD:6130XX21821_61304021821: WR-PHD 2.54 mm Dual Socket Header ARTICLE PROPERTIES: Pins:4;​ 6;​ 8;​ 10;​ 12;​ 14;​ 16;​ 18;​ 20;​ 22;​ 24;​ 26;​ 28;​ 30;​ 32;​ 34;​ 36;​ 40;​ 44;​ 64;​ 72 KIND PROPERTIES: Pitch：2.54 mm Quality Class:3 as per CECC 75 301-802 Rows：Dual Gender：Socket Header Type：Straight MATERIAL PROPERTIES: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; DATASHEET-URL: https://katalog.we-online.com/em/datasheet/61304021821.pdf; GENDER: Socket Header; IR: 3A; MATES: WR-PHD 2.54mm SMT Dual Pin Header/THT Angled Dual Pin Header/THT Dual Board Stacker/THT Dual Pin Header; PACKAGING: Tray; PART-NUMBER: 61304021821; PINS: 40; ROWS: Dual; TYPE: Straight
J3-J13 J15 J17 J19 J21 J23 = Wurth_Connectors_WR-PHD:6130XX11121_61300211121: WR-PHD 2.54 mm THT Pin Header; DATASHEET-URL: https://katalog.we-online.com/em/datasheet/61300211121.pdf; GENDER: Pin Header; IR: 3A; MATES: WR-PHD 2.54mm Angled Socket Header /SMT Socket Header/Socket Header; PACKAGING: Bag; PART-NUMBER: 61300211121; PINS: 2; ROWS: Single; TYPE: Straight
LED1 LED2 LED5 LED6 = adafruit:LED: LED
OK1-OK3 = optocoupler:HCPL2630: HEWLETT PACKARD OPTO COUPLER; MF: AGILENT TECHNOLOGIES; MPN: HCPL-2630-000E; OC_FARNELL: 9994904; OC_NEWARK: 88H7813
Q1-Q6 = transistor-power:IRFP25*: 33A/27A, 200V/150V, 0.085/0.012 Ohm, N-Channel Power MOSFET Source: Fairchild Semiconductor Corporation
R1-R69 R81 R85 R99-R101 R104-R106 R109-R131 R133-R135 R142 R144-R146 R149-R157 = rcl:R-EU_: RESISTOR, European symbol; SPICEPREFIX: R
SW1 = adafruit:SWITCH_PUSHBUTTON: Buttons
T1 T2 T7-T12 = transistor:BC547: NPN TRANSISTOR
U1-U3 U5 = IL300:IL300: Optoisolator Photovoltaic, Linearized Output 5300Vrms 1 Channel 8-SMD Check availability; AVAILABILITY: In Stock; DESCRIPTION: Optoisolator Photovoltaic, Linearized Output 5300Vrms 1 Channel 8-SMD; MF: Vishay; MP: IL300; PACKAGE: DIP-8 Vishay; PRICE: None; PURCHASE-URL: https://pricing.snapeda.com/search/part/IL300/?ref=eda
U4 U6 U7 = IR2183:IR2183: MOSFET DRVR 600V 2.3A 2-OUT Hi/Lo Side Half Brdg Inv/Non-Inv 8-Pin PDIP Check availability; AVAILABILITY: In Stock; DESCRIPTION: Half-Bridge Gate Driver IC Inverting, Non-Inverting 14-SOIC; MF: Infineon Technologies; MP: IR2183; PACKAGE: DIP-8 Infineon; PRICE: None; PURCHASE-URL: https://pricing.snapeda.com/search/part/IR2183/?ref=eda
U8-U14 = ACS722LLCTR-05AB-T:ACS722LLCTR-05AB-T: None Check availability; AVAILABILITY: In Stock; DESCRIPTION: Current Sensor 5A 1 Channel Hall Effect, Open Loop Bidirectional 8-SOIC (0.154, 3.90mm Width); MF: Allegro; MP: ACS722LLCTR-05AB-T; PACKAGE: SOIC-8 Allegro; PRICE: None
VR1-VR8 VR10 VR11 = 3296W-1-502LF:3296W-1-502LF: Res Cermet Trimmer 500K Ohm 10% 0.5W 25(Elec)Turn 2.19mm (9.53 X 4.83 X 11.55mm) Pin Thru-Hole Tube Check availability; AVAILABILITY: In Stock; DESCRIPTION: 5 kOhms 0.5W, 1/2W PC Pins Through Hole Trimmer Potentiometer Cermet 25.0 Turn Top Adjustment; MF: Bourns; MP: 3296W-1-502LF; PACKAGE: SOT-23-5 Bourns; PRICE: None; PURCHASE-URL: https://pricing.snapeda.com/search/part/3296W-1-502LF/?ref=eda
X1-X13 = con-phoenix-500:MSTBV2: PHOENIX; OC_FARNELL: unknown; OC_NEWARK: unknown

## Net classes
1 High_gnd: clearance 1 mm

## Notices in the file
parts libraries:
Wurth_Connectors_WR-PHD: Copyright: Würth Elektronik
